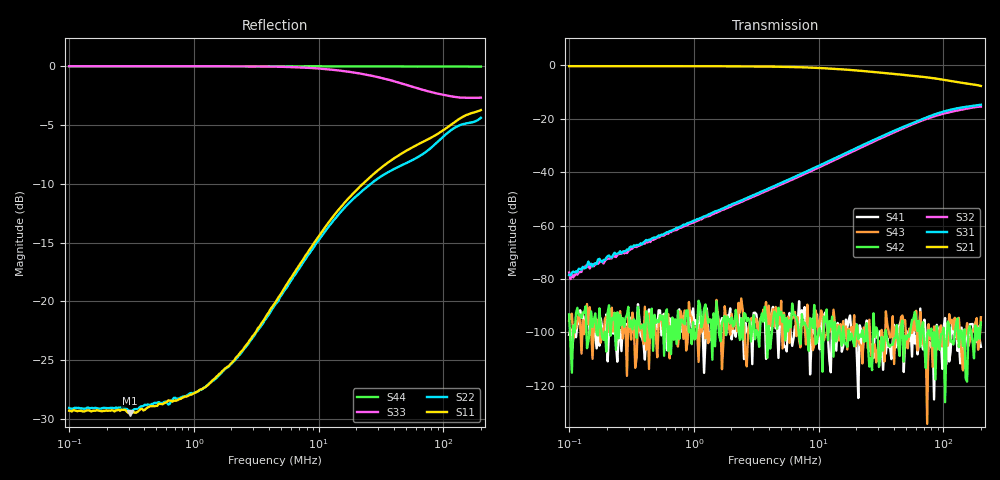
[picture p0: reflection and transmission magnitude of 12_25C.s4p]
!Keysight Technologies,E5080A,MY55200740,A.12.60.03
!Date: Friday, October 02, 2020 16:07:37
!Correction: S11(Full 4 Port(1,2,3,4))
!S12(Full 4 Port(1,2,3,4))
!S13(Full 4 Port(1,2,3,4))
!S14(Full 4 Port(1,2,3,4))
!S21(Full 4 Port(1,2,3,4))
!S22(Full 4 Port(1,2,3,4))
!S23(Full 4 Port(1,2,3,4))
!S24(Full 4 Port(1,2,3,4))
!S31(Full 4 Port(1,2,3,4))
!S32(Full 4 Port(1,2,3,4))
!S33(Full 4 Port(1,2,3,4))
!S34(Full 4 Port(1,2,3,4))
!S41(Full 4 Port(1,2,3,4))
!S42(Full 4 Port(1,2,3,4))
!S43(Full 4 Port(1,2,3,4))
!S44(Full 4 Port(1,2,3,4))
!S4P File: Measurements: <S11,S12,S13,S14>,
!<S21,S22,S23,S24>,
!<S31,S32,S33,S34>,
!<S41,S42,S43,S44>:Log Frequency Sweep
# Hz S  dB  R 50
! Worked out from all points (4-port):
!   300 points, 100 kHz to 200 MHz, reference 50 ohm
!   strongest paths, dB at 100 kHz, 673 kHz, 4.529 MHz, 30.48 MHz, 200 MHz:
!     S21: -0.3, -0.3, -0.5, -2.7, -7.7
!     S31: -78.5, -61.7, -44.9, -27.1, -14.7
!     S32: -77.6, -62.0, -45.5, -27.6, -15.4
!     S42: -93.3, -94.4, -92.9, -113.0, -96.3
!     S43: -95.6, -95.7, -90.5, -103.3, -94.3
!     S41: -100.9, -95.5, -98.5, -100.8, -105.4
!   lowest |S11| = -29.5 dB at 306 kHz (marker M1), VSWR 1.07, Z = 53.4 - j0.393 ohm
!   |S11| at or under -10 dB: start of sweep to 22.7 MHz
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100000  -29.30 -0.1  -0.31 -0.2  -79.08 101.6  -107.24 25.0
        -0.31 -0.1  -29.07 -0.1  -77.67 97.3  -90.84 178.8
        -78.47 91.8  -77.60 98.9  0.00 -0.1  -93.01 -25.8
        -100.89 -137.9  -93.27 19.0  -95.57 -116.6  0.00 -0.0
102574.7  -29.33 -0.4  -0.31 -0.2  -77.78 87.0  -96.79 166.3
          -0.31 -0.1  -29.13 -0.2  -77.60 93.1  -96.86 162.3
          -78.68 97.7  -80.04 83.9  -0.00 -0.1  -89.32 -10.4
          -98.67 -17.9  -104.43 -176.2  -93.46 -141.8  0.00 -0.0
306034.4  -29.53 -6.3  -0.31 -0.4  -68.81 92.0  -95.39 147.9
          -0.31 -0.4  -29.31 -5.6  -68.99 91.5  -95.72 110.4
          -68.13 92.9  -69.15 89.9  0.00 -0.4  -97.80 5.2
          -98.68 4.5  -98.01 -7.2  -95.67 77.3  0.00 -0.0
1908390  -25.52 -57.8  -0.34 -2.4  -52.63 90.8  -95.41 -138.0
         -0.34 -2.4  -25.53 -55.3  -53.10 90.8  -98.66 -141.8
         -52.47 90.9  -53.13 90.5  -0.01 -2.6  -96.72 -94.2
         -94.21 149.1  -95.39 -163.3  -98.21 -157.3  -0.00 -0.1
1.928983e7  -10.74 -123.9  -1.83 -14.0  -31.35 88.9  -100.21 61.3
            -1.84 -14.0  -11.22 -114.3  -31.93 91.4  -104.18 -24.6
            -31.34 88.7  -31.95 91.4  -0.54 -23.8  -99.41 84.4
            -99.39 -124.1  -105.19 -33.3  -93.56 177.4  -0.00 -1.3
7.612041e7  -6.19 -148.6  -4.56 -17.2  -19.20 62.7  -96.91 -151.4
            -4.56 -17.2  -7.12 -127.9  -19.78 70.4  -105.42 55.3
            -19.20 62.7  -19.78 70.5  -2.14 -69.1  -110.51 87.3
            -103.46 -127.9  -99.08 -84.7  -96.90 -86.8  -0.02 -5.2
2e8  -3.73 -160.4  -7.71 -11.2  -14.76 24.4  -104.50 -4.2
     -7.71 -11.2  -4.39 -107.9  -15.45 47.6  -99.98 134.2
     -14.74 24.5  -15.44 47.6  -2.67 -116.2  -93.97 -73.1
     -105.38 49.2  -96.30 148.5  -94.31 -50.1  -0.03 -13.5
